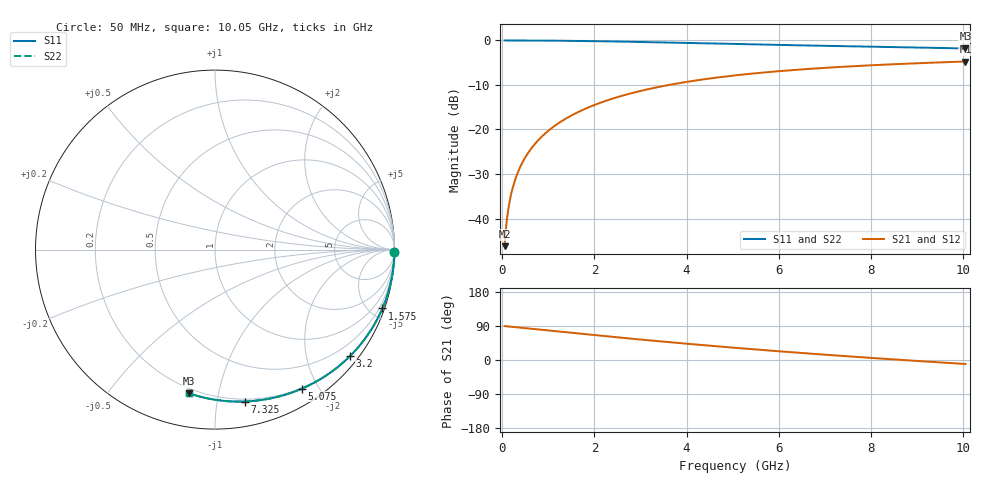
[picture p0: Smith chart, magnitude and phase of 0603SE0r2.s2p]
! AVX Thin Film Operation		Date: August 2001
! Description: Accu-P® Series, Thin Film, SMD, RF Capacitor
! Part Number: 06035J0R2ABT
! 50 MHz  -  10.05 GHz
! Serial Measurements
# mhz S db R 50
!	S11		S21		S12		S22
!	dB	Phase	dB	Phase	dB	Phase	dB	Phase
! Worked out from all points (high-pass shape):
!   401 points, 50 MHz to 10.05 GHz, reference 50 ohm
!   highest |S21| = -4.73 dB at 10.05 GHz (marker M1); lowest = -46.2 dB at 50 MHz (marker M2)
!   |S21| within 3 dB of the highest: 5.156 GHz to end of sweep
!   lowest |S11| = -1.8 dB at 10.05 GHz (marker M3), VSWR 9.71, Z = 8.66 - j40.9 ohm
!   |S11| at or under -10 dB: nowhere
!   |S22| runs from -1.8 to 0.0 dB; largest |S21 - S12| = 0
!   S11 on the Smith chart (normalised r, x): 50 MHz: open; 1.575 GHz: 0.20, -5.85; 3.2 GHz: 0.20, -2.87; 5.075 GHz: 0.19, -1.79; 7.325 GHz: 0.18, -1.20; 10.05 GHz: 0.17, -0.82
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50  -0.00 -0.6  -46.22 89.4  -46.22 89.4  -0.00 -0.6
75  -0.00 -0.9  -42.69 89.1  -42.69 89.1  -0.00 -0.9
125  -0.00 -1.6  -38.26 88.5  -38.26 88.5  -0.00 -1.6
150  -0.00 -1.9  -36.68 88.2  -36.68 88.2  -0.00 -1.9
225  -0.00 -2.8  -33.16 87.2  -33.16 87.2  -0.00 -2.8
325  -0.00 -4.0  -29.97 86.0  -29.97 86.0  -0.00 -4.0
475  -0.01 -5.9  -26.68 84.1  -26.68 84.1  -0.01 -5.9
675  -0.02 -8.4  -23.65 81.6  -23.65 81.6  -0.02 -8.4
925  -0.04 -11.4  -20.94 78.6  -20.94 78.6  -0.04 -11.4
1225  -0.06 -15.1  -18.55 74.9  -18.55 74.9  -0.06 -15.1
1575  -0.10 -19.4  -16.45 70.6  -16.45 70.6  -0.10 -19.4
1725  -0.12 -21.2  -15.70 68.8  -15.70 68.8  -0.12 -21.2
2400  -0.22 -29.2  -13.04 60.8  -13.04 60.8  -0.22 -29.1
3200  -0.37 -38.3  -10.87 51.7  -10.87 51.7  -0.37 -38.3
3400  -0.41 -40.5  -10.43 49.5  -10.43 49.5  -0.41 -40.5
4200  -0.59 -49.1  -8.99 40.9  -8.99 40.9  -0.59 -49.1
5050  -0.78 -57.8  -7.85 32.2  -7.85 32.2  -0.78 -57.8
5075  -0.79 -58.0  -7.82 31.9  -7.82 31.9  -0.79 -58.0
6725  -1.15 -73.5  -6.34 16.5  -6.34 16.5  -1.15 -73.5
7325  -1.28 -78.7  -5.95 11.2  -5.95 11.2  -1.28 -78.7
8400  -1.49 -87.6  -5.38 2.3  -5.38 2.3  -1.49 -87.6
10050  -1.80 -100.4  -4.73 -10.5  -4.73 -10.5  -1.80 -100.4
